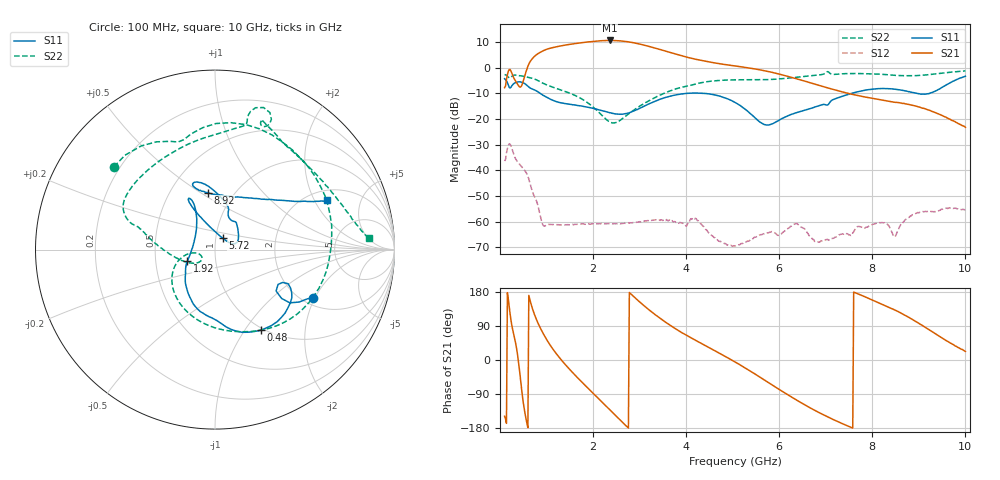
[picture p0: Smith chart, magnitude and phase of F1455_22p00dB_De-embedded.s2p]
! Integrated Device Technology
! Corporate Headquarters
! 6024 Silver Creek Valley Road
! San Jose, CA 95138  USA
! Phone:  1-408-284-8200
! Toll Free:  1-800-223-1366
! Webpage:  http://www.idt.com/
! Timing and RF Division
! 515 Groton Road, Suite 102
! Westford, MA 01886-6024
! Device:  F1455
! Description: 6-bit 0.5 dB Transmit Variable Gain Amplifier
! Frequency:  1400.0 -  2300.00 MHz
! Package:  6x6 mm Thin QFN Plastic Package: 28 pin
! State:  44
! Atten State:  22.0 dB
! Voltage:  +5.00 Volts
! Current:  217.634 mA
! Data:  The device was measured on a the F1455 evaluation board which has
!  individual transmission lines to the RF pins.  Data was collected
!  using a calibrated network analyzer.  The evaluation board was
!  de-embedded using a TRL calibration technique.
!  The reference plane is the edge of the package pin.
!  Pin  1 = CSb
!  Pin  2 = DATA
!  Pin  3 = CLK
!  Pin  4 = RSET
!  Pin  5 = GND
!  Pin  6 = RFIN  = Port 1
!  Pin  7 = GND
!  Pin  8 = NC
!  Pin  9 = NC
!  Pin 10 = NC
!  Pin 11 = NC
!  Pin 12 = NC
!  Pin 13 = NC
!  Pin 14 = /STBY
!  Pin 15 = GND
!  Pin 16 = RFOUT  = Port 2
!  Pin 17 = GND
!  Pin 18 = NC
!  Pin 19 = NC
!  Pin 20 = NC
!  Pin 21 = GND
!  Pin 22 = NC
!  Pin 23 = GND
!  Pin 24 = NC
!  Pin 25 = NC
!  Pin 26 = NC
!  Pin 27 = GND
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# GHz S dB R 50
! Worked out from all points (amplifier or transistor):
!   496 points, 100 MHz to 10 GHz, reference 50 ohm
!   highest |S21| = 10.6 dB at 2.36 GHz (marker M1)
!   |S21| within 3 dB of that: 1.086 GHz to 3.337 GHz (2.251 GHz wide, 102 % of centre)
!   unconditionally stable (mu >= 1): start of sweep to end of sweep
!   at 1.74 GHz: K = 165.21, MAG = 10.1 dB, |S12| = -60.9 dB
!   at 5.06 GHz: K = 874.61, MAG = 2.6 dB, |S12| = -69.4 dB
!   at 10 GHz: K = 577.41, MAG = -14.6 dB, |S12| = -55.3 dB
!   S11 on the Smith chart (normalised r, x): 100 MHz: 2.27, -1.93; 480 MHz: 0.97, -1.19; 1.92 GHz: 0.73, -0.10; 5.72 GHz: 1.08, +0.14; 8.92 GHz: 0.76, +0.54; 10 GHz: 2.45, +2.52
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0.1  -4.32 -26.1  -7.80 -148.4  -36.39 47.0  -2.76 140.7
0.18  -6.74 -36.2  -1.40 159.9  -30.27 -6.9  -3.69 112.6
0.26  -6.94 -25.0  -2.38 87.9  -31.77 -76.9  -3.32 95.9
0.38  -5.57 -42.2  -6.48 12.5  -36.72 -117.9  -3.01 58.0
0.48  -5.73 -60.4  -6.40 -92.7  -38.89 -149.5  -3.28 31.5
0.68  -8.22 -90.5  3.18 142.7  -47.30 138.3  -4.09 -15.8
0.82  -9.47 -108.9  5.49 96.6  -54.01 110.3  -5.07 -47.0
0.96  -11.13 -123.5  6.84 63.1  -61.72 126.6  -6.37 -72.3
1.34  -13.79 -143.4  8.59 -2.9  -61.20 101.1  -8.88 -122.3
1.76  -14.95 -153.4  9.73 -58.4  -60.86 69.9  -12.21 -156.9
1.92  -15.56 -157.0  10.08 -77.9  -60.89 61.0  -14.15 -165.8
2.36  -17.58 -176.4  10.59 -131.5  -60.77 44.0  -21.17 -160.8
2.78  -17.56 146.1  9.99 178.1  -60.59 35.3  -17.82 -144.4
3.08  -15.17 125.8  8.85 144.9  -59.97 28.2  -14.13 -162.3
3.4  -12.57 116.8  7.27 113.7  -59.25 16.1  -11.06 -178.9
4.08  -9.94 116.3  3.78 60.2  -59.47 4.0  -6.94 163.4
5.06  -13.63 114.8  0.64 -5.9  -69.43 2.6  -4.74 147.9
5.72  -22.35 56.4  -1.33 -55.7  -64.57 12.7  -4.67 120.9
6.7  -15.78 37.4  -6.07 -128.7  -66.44 -130.8  -3.13 78.4
8.36  -8.19 108.3  -13.14 138.7  -61.79 80.6  -2.78 62.2
8.92  -9.89 97.5  -14.90 102.7  -56.97 108.3  -3.11 39.7
10  -3.35 23.9  -23.25 22.6  -55.29 34.4  -1.28 4.4
